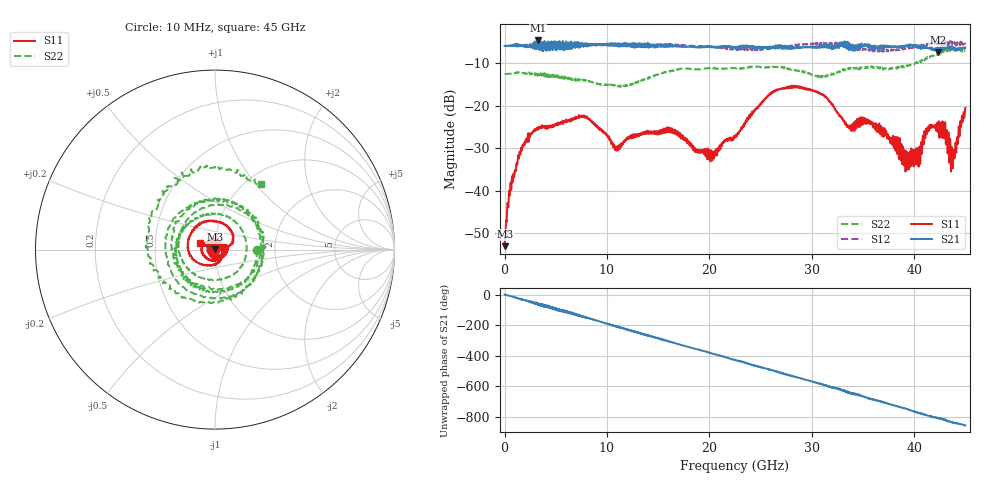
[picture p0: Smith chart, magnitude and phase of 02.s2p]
! 9/19/2025 2:50:19 PM
! C:\USERS\VECTORSTARUSER\DESKTOP\1942\02.S2P
! CHANNEL.1
! TR.MEASUREMENT
! CORRECTED.DATA
! RF.CORRECTION: FULL.TWO.PORT.CAL.PORT.1.2
! AVERAGING.OFF
! IF.BANDWIDTH: 1KHZ
! SWEEPTYPE:  FREQ.SWEEP(Linear)
! Reference Plane Port Info
! PORT:  PORT1  PORT2
! DISTANCE:  0  m  0  m
! TIME:  0  s  0  s
! PHASE.OFFSET:  0 °  0 °
! LOSS:  0  dB  0  dB
! REF.LOSS:  0  dB  0  dB
! REF.FREQ:  0  Hz  0  Hz
! Power Info
! POWER:  -10  dBm  -10  dBm
! EFF.POWER:  -10  dBm  -10  dBm
! SOURCE.ATTEN:  0  dB  0  dB
! TEST.ATTEN:  0  dB  0  dB
# GHZ S RI R 50.0
! FREQ.GHZ  S11RE  S11IM  S21RE  S21IM  S12RE  S12IM  S22RE  S22IM
!; PortSelection: Port_12
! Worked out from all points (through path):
!   1601 points, 10 MHz to 45 GHz, reference 50 ohm
!   highest |S21| = -4.71 dB at 3.272 GHz (marker M1); lowest = -7.5 dB at 42.3 GHz (marker M2)
!   group delay of S21, straight-line fit = 53 ps
!   lowest |S11| = -53.1 dB at 38.12 MHz (marker M3), VSWR 1.00, Z = 49.8 + j0.12 ohm
!   |S11| at or under -10 dB: start of sweep to end of sweep
!   |S22| runs from -15.6 to -6.6 dB; largest |S21 - S12| = 0.14
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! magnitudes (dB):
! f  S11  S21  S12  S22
! 10 MHz  -52.2  -6.0  -6.0  -12.6
! 38.12 MHz  -53.1  -6.0  -6.0  -12.6
! 516.1 MHz  -41.1  -6.1  -6.0  -12.5
! 1.388 GHz  -32.5  -5.9  -5.9  -12.2
! 3.272 GHz  -25.2  -4.7  -6.0  -12.5
! 7.518 GHz  -22.6  -6.0  -5.8  -14.0
! 10.92 GHz  -30.6  -5.7  -5.9  -15.3
! 15.03 GHz  -26.4  -5.8  -5.7  -12.7
! 20.11 GHz  -33.1  -6.0  -6.1  -11.1
! 22.5 GHz  -27.5  -6.3  -6.8  -11.2
! 26.27 GHz  -16.5  -6.4  -6.6  -11.0
! 30.01 GHz  -16.3  -6.2  -5.6  -12.8
! 33.64 GHz  -25.3  -6.5  -5.7  -11.1
! 35.27 GHz  -23.3  -5.9  -6.7  -10.9
! 37.52 GHz  -28.0  -6.0  -6.9  -11.5
! 39.35 GHz  -34.2  -6.1  -6.5  -10.7
! 40.44 GHz  -34.4  -6.2  -6.1  -9.7
! 41.51 GHz  -24.7  -6.3  -5.7  -8.6
! 42.3 GHz  -26.3  -7.5  -5.4  -7.8
! 42.95 GHz  -27.7  -6.6  -5.6  -7.1
! 43.79 GHz  -34.3  -6.8  -5.0  -6.6
! 45 GHz  -20.6  -6.4  -5.6  -7.0
